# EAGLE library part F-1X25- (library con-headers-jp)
FEMALE HEADER
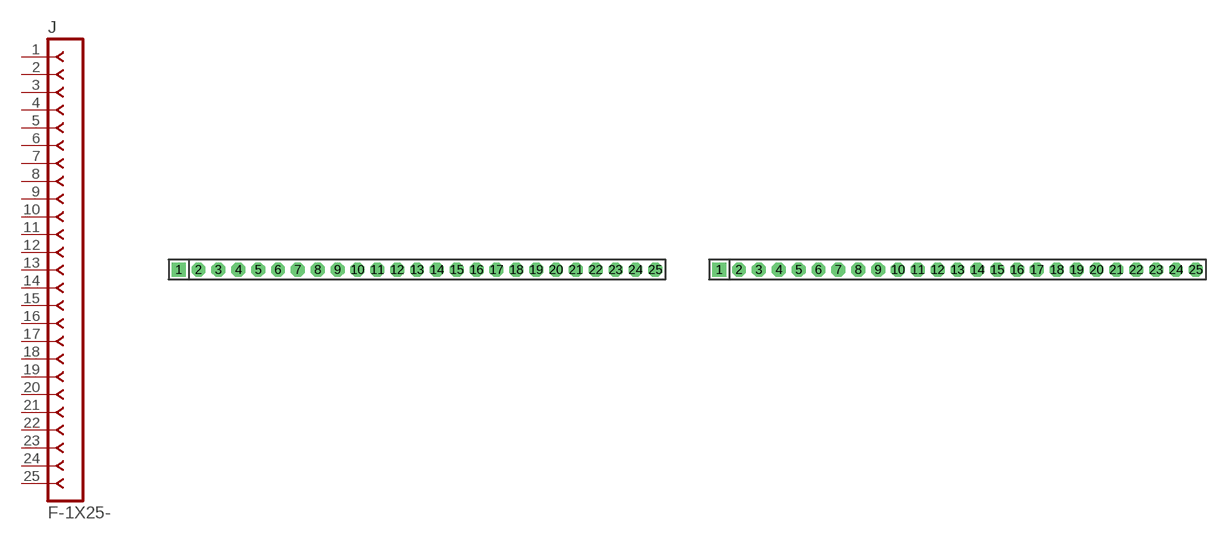
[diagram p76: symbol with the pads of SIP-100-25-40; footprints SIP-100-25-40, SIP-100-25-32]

Designator prefix J

## F-1X25-SIP-100-40  [SIP-100-25-40]
1  1  pas
2  2  pas
3  3  pas
4  4  pas
5  5  pas
6  6  pas
7  7  pas
8  8  pas
9  9  pas
10  10  pas
11  11  pas
12  12  pas
13  13  pas
14  14  pas
15  15  pas
16  16  pas
17  17  pas
18  18  pas
19  19  pas
20  20  pas
21  21  pas
22  22  pas
23  23  pas
24  24  pas
25  25  pas

## F-1X25-SIP-100-32  [SIP-100-25-32]
Pads as for SIP-100-25-40

## F-1X25-SIP-100-32Y  [SIP-100-25-32Y]
Pads as for SIP-100-25-40

## F-1X25-SIP-100-40Y  [SIP-100-25-40Y]
Pads as for SIP-100-25-40

## Footprint SIP-100-25-40 (pad centres in mm)
SIP Header - 0.1", 40 mil drill
drill 1.016 pad 1.778 square: 1 -30.48,0
drill 1.016 pad 1.778 octagon: 2 -27.94,0; 3 -25.4,0; 4 -22.86,0; 5 -20.32,0; 6 -17.78,0; 7 -15.24,0; 8 -12.7,0; 9 -10.16,0; 10 -7.62,0; 11 -5.08,0; 12 -2.54,0; 13 0,0; 14 2.54,0; 15 5.08,0; 16 7.62,0; 17 10.16,0; 18 12.7,0; 19 15.24,0; 20 17.78,0; 21 20.32,0; 22 22.86,0; 23 25.4,0; 24 27.94,0; 25 30.48,0

## Footprint SIP-100-25-32 (pad centres in mm)
SIP Header - 0.1", 32 mil drill
drill 0.813 pad 1.778 square: 1 -30.48,0
drill 0.813 pad 1.778 octagon: 2 -27.94,0; 3 -25.4,0; 4 -22.86,0; 5 -20.32,0; 6 -17.78,0; 7 -15.24,0; 8 -12.7,0; 9 -10.16,0; 10 -7.62,0; 11 -5.08,0; 12 -2.54,0; 13 0,0; 14 2.54,0; 15 5.08,0; 16 7.62,0; 17 10.16,0; 18 12.7,0; 19 15.24,0; 20 17.78,0; 21 20.32,0; 22 22.86,0; 23 25.4,0; 24 27.94,0; 25 30.48,0

## Footprint SIP-100-25-32Y (pad centres in mm)
SIP Header - 0.1", 32 mil drill
drill 0.813 long: 1 -30.48,0; 2 -27.94,0; 3 -25.4,0; 4 -22.86,0; 5 -20.32,0; 6 -17.78,0; 7 -15.24,0; 8 -12.7,0; 9 -10.16,0; 10 -7.62,0; 11 -5.08,0; 12 -2.54,0; 13 0,0; 14 2.54,0; 15 5.08,0; 16 7.62,0; 17 10.16,0; 18 12.7,0; 19 15.24,0; 20 17.78,0; 21 20.32,0; 22 22.86,0; 23 25.4,0; 24 27.94,0; 25 30.48,0

## Footprint SIP-100-25-40Y (pad centres in mm)
SIP Header - 0.1", 40 mil drill
drill 1.016 long: 1 -30.48,0; 2 -27.94,0; 3 -25.4,0; 4 -22.86,0; 5 -20.32,0; 6 -17.78,0; 7 -15.24,0; 8 -12.7,0; 9 -10.16,0; 10 -7.62,0; 11 -5.08,0; 12 -2.54,0; 13 0,0; 14 2.54,0; 15 5.08,0; 16 7.62,0; 17 10.16,0; 18 12.7,0; 19 15.24,0; 20 17.78,0; 21 20.32,0; 22 22.86,0; 23 25.4,0; 24 27.94,0; 25 30.48,0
